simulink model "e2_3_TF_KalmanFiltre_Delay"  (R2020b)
settings: Solver=ode4  StartTime=0.0  StopTime=100  FixedStep=sampleTime  RelTol=1e-3  EnableMultiTasking=on
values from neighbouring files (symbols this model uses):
  k_d_x = 0.7    [startSimulation.m]
  k_d_y = 0.7    [startSimulation.m]
  k_d_yaw = 0.05    [startSimulation.m]
  k_d_z = 0.05    [startSimulation.m]
  k_i_x = 0.01    [startSimulation.m]
  k_i_y = 0.01    [startSimulation.m]
  k_i_yaw = 0.01    [startSimulation.m]
  k_i_z = 0.01    [startSimulation.m]
  k_p_x = 1    [startSimulation.m]
  k_p_y = 1    [startSimulation.m]
  k_p_yaw = 2    [startSimulation.m]
  k_p_z = 3    [startSimulation.m]
  saturation_psi = 2    [startSimulation.m]
  saturation_x = 2    [startSimulation.m]
  saturation_y = 2    [startSimulation.m]
  saturation_z = 2    [startSimulation.m]
undefined symbols (not defined in the file or in its folder): DiscIntNeverNeededParam, KiRollAttitude, sigbuilder_block
libraries: simulink x7, pid_lib x2, aerolibanimutils x1

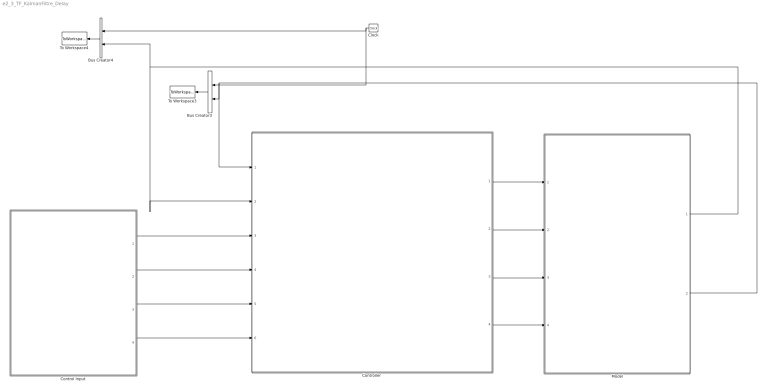
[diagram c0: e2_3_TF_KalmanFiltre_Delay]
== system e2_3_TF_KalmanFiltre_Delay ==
  Bus Creator3 : BusCreator  Inputs=2
  Bus Creator4 : BusCreator  Inputs=2
  Clock : Clock
  Control Input : Subsystem
  "Controller " : Subsystem
  Model : Subsystem
  To Workspace3 : ToWorkspace  VariableName=r1_pos_array  SampleTime=-1
  To Workspace4 : ToWorkspace  VariableName=r1_vel_array  SampleTime=-1
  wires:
  Clock/1 -> Bus Creator4/1, Bus Creator3/1
  Bus Creator3/1 -> To Workspace3/1
  Bus Creator4/1 -> To Workspace4/1
  "Controller "/1(Controller Output X) -> Model/1(Commande Input X)
  "Controller "/2(Controller Output Y) -> Model/2(Commande Input Y)
  "Controller "/3(Controller Output H) -> Model/3(Commande Input H)
  "Controller "/4(Controller Output Psi) -> Model/4(Commande Input Psi)
  Control Input/1(ux) -> "Controller "/3(Control input X)
  Control Input/2(uy) -> "Controller "/4(Control input Y)
  Control Input/3(uz) -> "Controller "/5(Control input H)
  Control Input/4(upsi) -> "Controller "/6(Control input Psi)
  Model/2(Output Position) -> "Controller "/1(Feedback Position), Bus Creator3/2
  Model/1(Output Velocity) -> "Controller "/2(Feedback Velocity), Bus Creator4/2

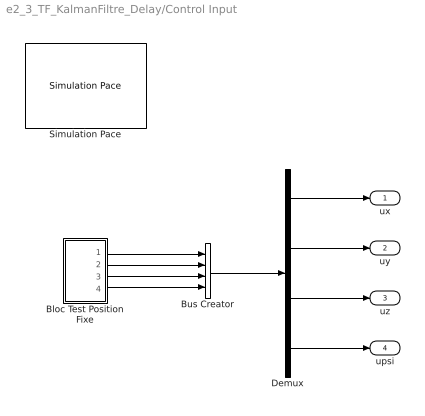
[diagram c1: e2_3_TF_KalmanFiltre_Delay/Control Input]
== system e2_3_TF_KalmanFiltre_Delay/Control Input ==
  Bloc Test Position Fixe : Subsystem
  Bus Creator : BusCreator  Inputs=4
  Demux : Demux
  Simulation Pace : aerolibanimutils/Simulation Pace  SimulationPace=100  SleepMode=MATLAB Thread  OutputPaceError=off  SampleTime=-1
  ux : Outport  VectorParamsAs1DForOutWhenUnconnected=off
  uy : Outport  Port=2  VectorParamsAs1DForOutWhenUnconnected=off
  uz : Outport  Port=3  VectorParamsAs1DForOutWhenUnconnected=off
  upsi : Outport  Port=4  VectorParamsAs1DForOutWhenUnconnected=off
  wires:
  Demux/2 -> uy/1
  Demux/1 -> ux/1
  Bloc Test Position Fixe/2(uy) -> Bus Creator/2
  Demux/3 -> uz/1
  Demux/4 -> upsi/1
  Bloc Test Position Fixe/4(upsi) -> Bus Creator/4
  Bloc Test Position Fixe/3(uz) -> Bus Creator/3
  Bloc Test Position Fixe/1(ux) -> Bus Creator/1
  Bus Creator/1 -> Demux/1

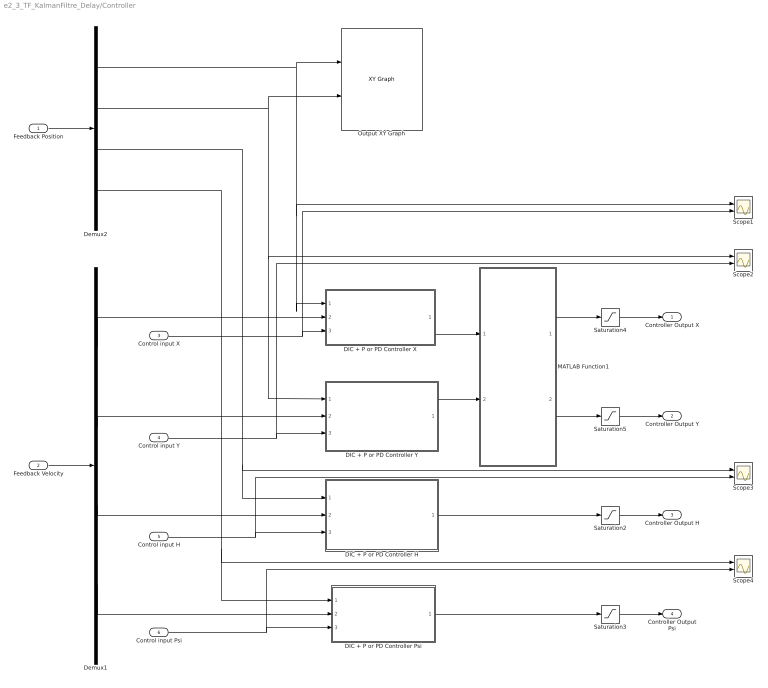
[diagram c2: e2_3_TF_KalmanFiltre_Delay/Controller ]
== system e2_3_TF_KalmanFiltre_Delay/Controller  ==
  Feedback Position : Inport
  Feedback Velocity : Inport  Port=2
  Control input X : Inport  Port=3
  Control input Y : Inport  Port=4
  Control input H : Inport  Port=5
  Control input Psi : Inport  Port=6
  DIC + P or PD Controller H : Subsystem
  DIC + P or PD Controller Psi : Subsystem
  DIC + P or PD Controller X : Subsystem
  DIC + P or PD Controller Y : Subsystem
  Demux1 : Demux
  Demux2 : Demux
  MATLAB Function1 : MATLAB Function  TreatAsAtomicUnit=on
  Output XY Graph : simulink/Sinks/XY Graph  Commented=on  xmin=-5  xmax=5  ymin=-5  ymax=5  st=-1
  Saturation2 : Saturate  UpperLimit=saturation_z  LowerLimit=-saturation_z
  Saturation3 : Saturate  UpperLimit=saturation_psi  LowerLimit=-saturation_psi
  Saturation4 : Saturate  UpperLimit=saturation_x  LowerLimit=-saturation_x
  Saturation5 : Saturate  UpperLimit=saturation_y  LowerLimit=-saturation_y
  Scope{1..4} (4 alike) : Scope  NumInputPorts=2
  Controller Output X : Outport  VectorParamsAs1DForOutWhenUnconnected=off
  Controller Output Y : Outport  Port=2  VectorParamsAs1DForOutWhenUnconnected=off
  Controller Output H : Outport  Port=3  VectorParamsAs1DForOutWhenUnconnected=off
  Controller Output Psi : Outport  Port=4  VectorParamsAs1DForOutWhenUnconnected=off
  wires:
  Feedback Position/1 -> Demux2/1
  Feedback Velocity/1 -> Demux1/1
  Demux1/2 -> DIC + P or PD Controller Y/2(Feedback Velocity Y)
  Demux2/3 -> Scope3/1, DIC + P or PD Controller H/1(Feedback Position H)
  Demux1/1 -> DIC + P or PD Controller X/2(Feedback Velocity X)
  Demux1/3 -> DIC + P or PD Controller H/2(Feedback Velocity H)
  Control input X/1 -> Scope1/2, DIC + P or PD Controller X/3(Control Input X)
  Control input H/1 -> Scope3/2, DIC + P or PD Controller H/3(Control Input H)
  Saturation4/1 -> Controller Output X/1
  Saturation5/1 -> Controller Output Y/1
  Saturation2/1 -> Controller Output H/1
  Saturation3/1 -> Controller Output Psi/1
  Control input Y/1 -> Scope2/2, DIC + P or PD Controller Y/3(Control Input Y)
  DIC + P or PD Controller H/1(Controller Output H) -> Saturation2/1
  DIC + P or PD Controller Psi/1(Controller Output Psi) -> Saturation3/1
  Demux2/1 -> Scope1/1, DIC + P or PD Controller X/1(Feedback Position X), Output XY Graph/1
  Demux2/2 -> Scope2/1, DIC + P or PD Controller Y/1(Feedback Position Y), Output XY Graph/2
  Demux2/4 -> Scope4/1, DIC + P or PD Controller Psi/1(Feedback Position Psi)
  Demux1/4 -> DIC + P or PD Controller Psi/2(Feedback Velocity Psi)
  Control input Psi/1 -> Scope4/2, DIC + P or PD Controller Psi/3(Control input Psi)
  MATLAB Function1/2(phi) -> Saturation5/1
  MATLAB Function1/1(theta) -> Saturation4/1
  DIC + P or PD Controller X/1(Controller Output X) -> MATLAB Function1/1(eax)
  DIC + P or PD Controller Y/1(Controller Output Y) -> MATLAB Function1/2(eay)

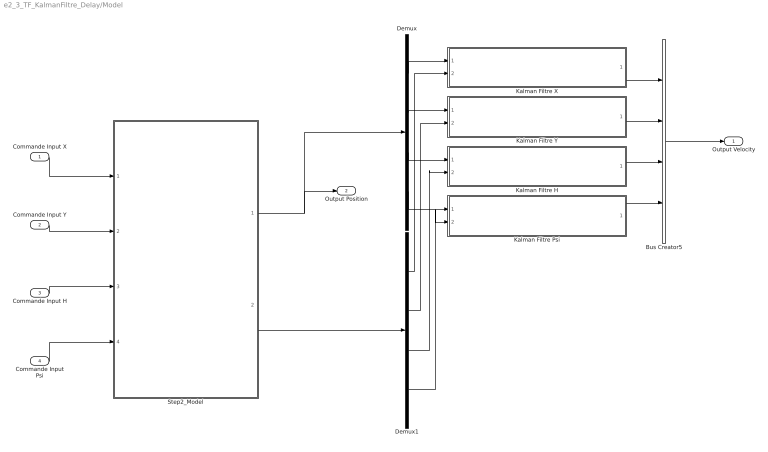
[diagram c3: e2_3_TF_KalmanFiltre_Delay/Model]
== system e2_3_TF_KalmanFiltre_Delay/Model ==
  Commande Input X : Inport
  Commande Input Y : Inport  Port=2
  Commande Input H : Inport  Port=3
  Commande Input Psi : Inport  Port=4
  Bus Creator5 : BusCreator  Inputs=4
  Demux : Demux
  Demux1 : Demux
  Kalman Filtre H : Subsystem
  Kalman Filtre Psi : Subsystem
  Kalman Filtre X : Subsystem
  Kalman Filtre Y : Subsystem
  Step2_Model : Subsystem
  Output Velocity : Outport  VectorParamsAs1DForOutWhenUnconnected=off
  Output Position : Outport  Port=2  VectorParamsAs1DForOutWhenUnconnected=off
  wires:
  Demux/4 -> Kalman Filtre Psi/1(The system output: Position)
  Bus Creator5/1 -> Output Velocity/1
  Demux/1 -> Kalman Filtre X/1(The system output: Position)
  Kalman Filtre X/1(Out velocity feedback) -> Bus Creator5/1
  Kalman Filtre Psi/1(Out velocity feedback) -> Bus Creator5/4
  Demux/2 -> Kalman Filtre Y/1(The system output: Position)
  Kalman Filtre Y/1(Out velocity feedback) -> Bus Creator5/2
  Kalman Filtre H/1(Out velocity feedback) -> Bus Creator5/3
  Demux/3 -> Kalman Filtre H/1(The system output: Position)
  Demux1/1 -> Kalman Filtre X/2(In2)
  Demux1/2 -> Kalman Filtre Y/2(In2)
  Demux1/3 -> Kalman Filtre H/2(In2)
  Demux1/4 -> Kalman Filtre Psi/2(In2)
  Commande Input H/1 -> Step2_Model/3(In3)
  Step2_Model/1(Position) -> Output Position/1, Demux/1
  Commande Input Psi/1 -> Step2_Model/4(In4)
  Commande Input X/1 -> Step2_Model/1(In1)
  Commande Input Y/1 -> Step2_Model/2(In2)
  Step2_Model/2(Velocity) -> Demux1/1

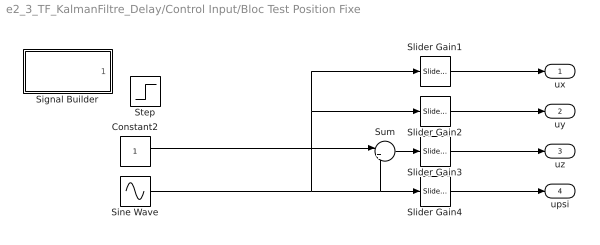
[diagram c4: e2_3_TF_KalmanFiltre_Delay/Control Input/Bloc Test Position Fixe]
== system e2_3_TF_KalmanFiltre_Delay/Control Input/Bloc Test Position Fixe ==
  Constant2 : Constant
  Signal Builder : Subsystem  Tag=STV Subsys  LoadFcn=sigbuilder_block('load');  StartFcn=sigbuilder_block('start');  StopFcn=sigbuilder_block('stop');  ClipboardFcn=sigbuilder_block('clipboard');  mask(Sigbuilder block){tuvar=[0:10]}
      mask help: Simulink:masks:SigbuilderBlock_MD
      mask init:
      | if ~strcmp(get_param(bdroot(gcbh),'SimulationStatus'),'stopped') tuvar = sigbuilder_block('maskInit'); end
  Sine Wave : Sin  Frequency=0.5  SampleTime=0
  Slider Gain1 : simulink/Math Operations/Slider Gain  gain=1  low=-10  high=10
  Slider Gain2 : simulink/Math Operations/Slider Gain  gain=0  low=-10  high=10
  Slider Gain3 : simulink/Math Operations/Slider Gain  gain=1  low=-2  high=2
  Slider Gain4 : simulink/Math Operations/Slider Gain  gain=0  low=-2  high=2
  Step : Step  Time=5  SampleTime=0
  Sum : Sum  Inputs=|++
  ux : Outport  VectorParamsAs1DForOutWhenUnconnected=off
  uy : Outport  Port=2  VectorParamsAs1DForOutWhenUnconnected=off
  uz : Outport  Port=3  VectorParamsAs1DForOutWhenUnconnected=off
  upsi : Outport  Port=4  VectorParamsAs1DForOutWhenUnconnected=off
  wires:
  Slider Gain1/1 -> ux/1
  Slider Gain2/1 -> uy/1
  Slider Gain3/1 -> uz/1
  Slider Gain4/1 -> upsi/1
  Sum/1 -> Slider Gain3/1
  Constant2/1 -> Sum/1
  Sine Wave/1 -> Slider Gain2/1, Slider Gain1/1, Sum/2, Slider Gain4/1

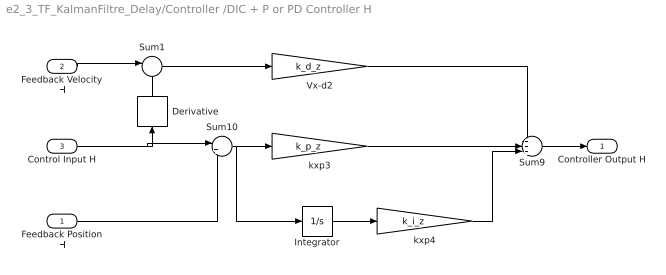
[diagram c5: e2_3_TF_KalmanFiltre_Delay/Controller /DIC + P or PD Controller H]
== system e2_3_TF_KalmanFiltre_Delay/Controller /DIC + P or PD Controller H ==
  Feedback Position H : Inport
  Feedback Velocity H : Inport  Port=2
  Control Input H : Inport  Port=3
  Derivative : Derivative
  Integrator : Integrator
  Sum1 : Sum  Inputs=|-+
  Sum10 : Sum  Inputs=|+-
  Sum9 : Sum  Inputs=+++|
  Vx-d2 : Gain  Gain=k_d_z
  kxp3 : Gain  Gain=k_p_z
  kxp4 : Gain  Gain=k_i_z
  Controller Output H : Outport  VectorParamsAs1DForOutWhenUnconnected=off
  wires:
  Sum9/1 -> Controller Output H/1
  Sum10/1 -> kxp3/1, Integrator/1
  kxp3/1 -> Sum9/2
  Vx-d2/1 -> Sum9/1
  Feedback Velocity H/1 -> Sum1/1
  Sum1/1 -> Vx-d2/1
  Integrator/1 -> kxp4/1
  kxp4/1 -> Sum9/3
  Control Input H/1 -> Sum10/1, Derivative/1
  Feedback Position H/1 -> Sum10/2
  Derivative/1 -> Sum1/2

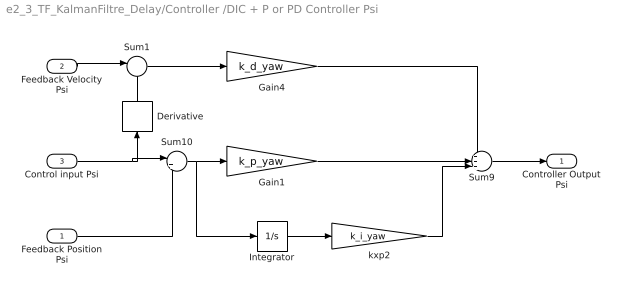
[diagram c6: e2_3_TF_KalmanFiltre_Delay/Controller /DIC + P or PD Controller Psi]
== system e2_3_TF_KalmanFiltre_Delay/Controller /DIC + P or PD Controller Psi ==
  Feedback Position Psi : Inport
  Feedback Velocity Psi : Inport  Port=2
  Control input Psi : Inport  Port=3
  Derivative : Derivative
  Gain1 : Gain  Gain=k_p_yaw
  Gain4 : Gain  Gain=k_d_yaw
  Integrator : Integrator
  Sum1 : Sum  Inputs=|-+
  Sum10 : Sum  Inputs=|+-
  Sum9 : Sum  Inputs=+++|
  kxp2 : Gain  Gain=k_i_yaw
  Controller Output Psi : Outport  VectorParamsAs1DForOutWhenUnconnected=off
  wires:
  Sum9/1 -> Controller Output Psi/1
  kxp2/1 -> Sum9/3
  Control input Psi/1 -> Sum10/1, Derivative/1
  Gain4/1 -> Sum9/1
  Sum10/1 -> Gain1/1, Integrator/1
  Integrator/1 -> kxp2/1
  Feedback Velocity Psi/1 -> Sum1/1
  Sum1/1 -> Gain4/1
  Gain1/1 -> Sum9/2
  Derivative/1 -> Sum1/2
  Feedback Position Psi/1 -> Sum10/2

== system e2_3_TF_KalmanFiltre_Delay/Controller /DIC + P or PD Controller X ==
  Feedback Position X : Inport
  Feedback Velocity X : Inport  Port=2
  Control Input X : Inport  Port=3
  PID1 : Subsystem
  Sum3 : Sum  Inputs=|+-
  Sum4 : Sum  Inputs=|+-
  roll_attitude2 : pid_lib/PID Controller  Controller=P  Form=Parallel  TimeDomain=Discrete-time  UseExternalTs=off  SampleTime=-1  IntegratorMethod=Forward Euler  FilterMethod=Forward Euler  ControllerParametersSource=internal  P=1  I=KiRollAttitude  D=0.01  UseFilter=on  N=100  TunerSelectOption=Transfer Function Based (PID Tuner App)  InitialConditionSource=internal  InitialConditionForIntegrator=0  InitialConditionForFilter=0  DifferentiatorICPrevScaledInput=0  ExternalReset=none  TrackingMode=off  Kt=1  LimitOutput=on  SatLimitsSource=internal  UpperSaturationLimit=100  LowerSaturationLimit=-100  LinearizeAsGain=on  AntiWindupMode=back-calculation  Kb=1  POutMin=[]  POutMax=[]  IOutMin=[]  IOutMax=[]  DOutMin=[]  DOutMax=[]  NOutMin=[]  NOutMax=[]  SumOutMin=[]  SumOutMax=[]  SaturationOutMin=[]  SaturationOutMax=[]  PParamMin=[]  PParamMax=[]  IParamMin=[]  IParamMax=[]  DParamMin=[]  DParamMax=[]  NParamMin=[]  NParamMax=[]  KbParamMin=[]  KbParamMax=[]  KtParamMin=[]  KtParamMax=[]  KbOutMin=[]  KbOutMax=[]  KtOutMin=[]  KtOutMax=[]  IntegratorOutMin=[]  IntegratorOutMax=[]  FilterOutMin=[]  FilterOutMax=[]  SumI1OutMin=[]  SumI1OutMax=[]  SumI2OutMin=[]  SumI2OutMax=[]  SumI3OutMin=[]  SumI3OutMax=[]  SumI4OutMin=[]  SumI4OutMax=[]  SumDOutMin=[]  SumDOutMax=[]  DifferentiatorOutMin=[]  DifferentiatorOutMax=[]  FilterDiffOutCoefMin=[]  FilterDiffOutCoefMax=[]  ReciprocalOutMin=[]  ReciprocalOutMax=[]  SumDenOutMin=[]  SumDenOutMax=[]  SumNumOutMin=[]  SumNumOutMax=[]  DivideOutMin=[]  DivideOutMax=[]  UdiffTsProdOutMin=[]  UdiffTsProdOutMax=[]  NTsProdOutMin=[]  NTsProdOutMax=[]  UintegralTsProdOutMin=[]  UintegralTsProdOutMax=[]  UngainTsProdOutMin=[]  UngainTsProdOutMax=[]  IntegratorContinuousStateAttributes=''  IntegratorStateMustResolveToSignalObject=off  IntegratorRTWStateStorageClass=Auto  FilterContinuousStateAttributes=''  FilterStateMustResolveToSignalObject=off  FilterRTWStateStorageClass=Auto  ParallelPVariant=InternalParameters  IdealPVariant=Disabled  IVariant=Disabled  DVariant=Disabled  IntegratorVariant=Disabled  SatVariant=Enabled  AWVariant=Disabled  PCopyVariant=Disabled  TRVariant=Disabled  FdbkBlocksVariant=Forward  IdealPFdbkVariant=Disabled  SatFdbkVariant=Disabled  DerivativeFilterVariant=Disabled  NVariant=Disabled  NCopyVariant=Disabled_SignalSpec  FilterICVariant=Disabled  IntegratorICVariant=Disabled  ExternalResetVariant=Disabled  TRSumVariant=Passthrough  SumFdbkVariant=Disabled  SumVariant=Passthrough_P  TsampFilterVariant=InternalTs  TsampNgainVariant=Passthrough  TsampIntegralVariant=Disabled_SignalSpec  ExternalSaturationOutDataTypeStr=Inherit: Same as second input
  Controller Output X : Outport  VectorParamsAs1DForOutWhenUnconnected=off
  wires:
  roll_attitude2/1 -> Sum4/1
  Sum3/1 -> roll_attitude2/1
  Sum4/1 -> PID1/1(x)
  PID1/1(y) -> Controller Output X/1
  Feedback Velocity X/1 -> Sum4/2
  Control Input X/1 -> Sum3/1
  Feedback Position X/1 -> Sum3/2

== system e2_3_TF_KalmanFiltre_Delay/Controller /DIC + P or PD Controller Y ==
  Feedback Position Y : Inport
  Feedback Velocity Y : Inport  Port=2
  Control Input Y : Inport  Port=3
  PID2 : Subsystem
  Sum : Sum  Inputs=|+-
  Sum2 : Sum  Inputs=|+-
  roll_attitude : pid_lib/PID Controller  Controller=P  Form=Parallel  TimeDomain=Discrete-time  UseExternalTs=off  SampleTime=-1  IntegratorMethod=Forward Euler  FilterMethod=Forward Euler  ControllerParametersSource=internal  P=1  I=KiRollAttitude  D=0.01  UseFilter=on  N=100  TunerSelectOption=Transfer Function Based (PID Tuner App)  InitialConditionSource=internal  InitialConditionForIntegrator=0  InitialConditionForFilter=0  DifferentiatorICPrevScaledInput=0  ExternalReset=none  TrackingMode=off  Kt=1  LimitOutput=on  SatLimitsSource=internal  UpperSaturationLimit=1  LowerSaturationLimit=-1  LinearizeAsGain=on  AntiWindupMode=back-calculation  Kb=1  POutMin=[]  POutMax=[]  IOutMin=[]  IOutMax=[]  DOutMin=[]  DOutMax=[]  NOutMin=[]  NOutMax=[]  SumOutMin=[]  SumOutMax=[]  SaturationOutMin=[]  SaturationOutMax=[]  PParamMin=[]  PParamMax=[]  IParamMin=[]  IParamMax=[]  DParamMin=[]  DParamMax=[]  NParamMin=[]  NParamMax=[]  KbParamMin=[]  KbParamMax=[]  KtParamMin=[]  KtParamMax=[]  KbOutMin=[]  KbOutMax=[]  KtOutMin=[]  KtOutMax=[]  IntegratorOutMin=[]  IntegratorOutMax=[]  FilterOutMin=[]  FilterOutMax=[]  SumI1OutMin=[]  SumI1OutMax=[]  SumI2OutMin=[]  SumI2OutMax=[]  SumI3OutMin=[]  SumI3OutMax=[]  SumI4OutMin=[]  SumI4OutMax=[]  SumDOutMin=[]  SumDOutMax=[]  DifferentiatorOutMin=[]  DifferentiatorOutMax=[]  FilterDiffOutCoefMin=[]  FilterDiffOutCoefMax=[]  ReciprocalOutMin=[]  ReciprocalOutMax=[]  SumDenOutMin=[]  SumDenOutMax=[]  SumNumOutMin=[]  SumNumOutMax=[]  DivideOutMin=[]  DivideOutMax=[]  UdiffTsProdOutMin=[]  UdiffTsProdOutMax=[]  NTsProdOutMin=[]  NTsProdOutMax=[]  UintegralTsProdOutMin=[]  UintegralTsProdOutMax=[]  UngainTsProdOutMin=[]  UngainTsProdOutMax=[]  IntegratorContinuousStateAttributes=''  IntegratorStateMustResolveToSignalObject=off  IntegratorRTWStateStorageClass=Auto  FilterContinuousStateAttributes=''  FilterStateMustResolveToSignalObject=off  FilterRTWStateStorageClass=Auto  ParallelPVariant=InternalParameters  IdealPVariant=Disabled  IVariant=Disabled  DVariant=Disabled  IntegratorVariant=Disabled  SatVariant=Enabled  AWVariant=Disabled  PCopyVariant=Disabled  TRVariant=Disabled  FdbkBlocksVariant=Forward  IdealPFdbkVariant=Disabled  SatFdbkVariant=Disabled  DerivativeFilterVariant=Disabled  NVariant=Disabled  NCopyVariant=Disabled_SignalSpec  FilterICVariant=Disabled  IntegratorICVariant=Disabled  ExternalResetVariant=Disabled  TRSumVariant=Passthrough  SumFdbkVariant=Disabled  SumVariant=Passthrough_P  TsampFilterVariant=InternalTs  TsampNgainVariant=Passthrough  TsampIntegralVariant=Disabled_SignalSpec  ExternalSaturationOutDataTypeStr=Inherit: Same as second input
  Controller Output Y : Outport  VectorParamsAs1DForOutWhenUnconnected=off
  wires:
  Sum/1 -> roll_attitude/1
  roll_attitude/1 -> Sum2/1
  Sum2/1 -> PID2/1(x)
  Feedback Position Y/1 -> Sum/2
  Feedback Velocity Y/1 -> Sum2/2
  Control Input Y/1 -> Sum/1
  PID2/1(y) -> Controller Output Y/1

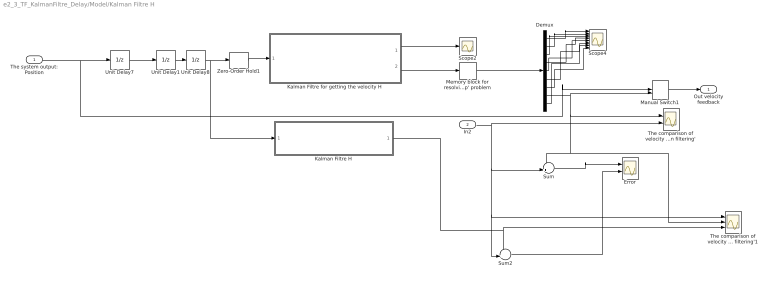
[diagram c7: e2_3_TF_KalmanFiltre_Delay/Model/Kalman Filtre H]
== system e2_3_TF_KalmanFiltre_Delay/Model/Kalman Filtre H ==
  The system output: Position : Inport
  In2 : Inport  Port=2
  Demux : Demux  Outputs=9
  Error : Scope  NumInputPorts=2
  Kalman Filtre H : Subsystem
  Kalman Filtre for getting the velocity H : MATLAB Function  TreatAsAtomicUnit=on  SystemSampleTime=0.01
  Manual Switch1 : ManualSwitch  CurrentSetting=0
  Memory block for resolving the 'algebraic loop' problem : Memory
  Scope2 : Scope
  Scope4 : Scope  NumInputPorts=8
  Sum : Sum  Inputs=-+|
  Sum2 : Sum  Inputs=-+|
  The comparison of velocity signal between 'Derivative' and 'Kalman filtering' : Scope  NumInputPorts=2
  The comparison of velocity signal between 'Derivative' and 'Kalman filtering'1 : Scope  NumInputPorts=3
  Unit Delay1 : UnitDelay  SampleTime=-1  HasFrameUpgradeWarning=on
  Unit Delay7 : UnitDelay  SampleTime=-1  HasFrameUpgradeWarning=on
  Unit Delay8 : UnitDelay  SampleTime=-1  HasFrameUpgradeWarning=on
  Zero-Order Hold1 : ZeroOrderHold  SampleTime=-1
  Out velocity feedback : Outport  VectorParamsAs1DForOutWhenUnconnected=off
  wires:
  Kalman Filtre for getting the velocity H/1(Covariance_matrice) -> Scope2/1
  Kalman Filtre for getting the velocity H/2(X_Kalmanfiltred) -> Memory block for resolving the 'algebraic loop' problem/1
  Memory block for resolving the 'algebraic loop' problem/1 -> Demux/1
  Zero-Order Hold1/1 -> Kalman Filtre for getting the velocity H/1(Mesurement_Velocity)
  Manual Switch1/1 -> Out velocity feedback/1
  Demux/1 -> Scope4/1
  The system output: Position/1 -> Unit Delay7/1, Manual Switch1/1
  Demux/2 -> Scope4/2
  Demux/3 -> Scope4/3
  Demux/4 -> Scope4/4
  Demux/5 -> Scope4/5
  Unit Delay8/1 -> Kalman Filtre H/1(The system output: Position), Zero-Order Hold1/1
  Demux/6 -> Scope4/6
  Demux/7 -> Scope4/8
  Demux/8 -> The comparison of velocity signal between 'Derivative' and 'Kalman filtering'1/2, Sum/1, The comparison of velocity signal between 'Derivative' and 'Kalman filtering'/1, Manual Switch1/2
  Demux/9 -> Scope4/7
  In2/1 -> The comparison of velocity signal between 'Derivative' and 'Kalman filtering'/2, Sum2/2, The comparison of velocity signal between 'Derivative' and 'Kalman filtering'1/1, Sum/2
  Unit Delay7/1 -> Unit Delay1/1
  Unit Delay1/1 -> Unit Delay8/1
  Sum/1 -> Error/1
  Kalman Filtre H/1(Out velocity feedback) -> Sum2/1, The comparison of velocity signal between 'Derivative' and 'Kalman filtering'1/3
  Sum2/1 -> Error/2

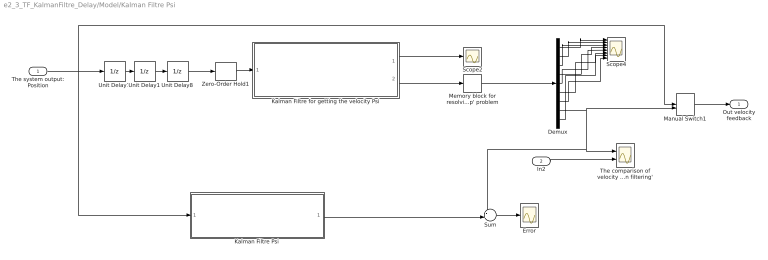
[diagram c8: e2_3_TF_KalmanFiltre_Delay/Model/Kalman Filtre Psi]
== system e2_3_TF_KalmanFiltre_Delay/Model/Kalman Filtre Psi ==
  The system output: Position : Inport
  In2 : Inport  Port=2
  Demux : Demux  Outputs=9
  Error : Scope
  Kalman Filtre Psi : Subsystem
  Kalman Filtre for getting the velocity Psi : MATLAB Function  TreatAsAtomicUnit=on  SystemSampleTime=0.01
  Manual Switch1 : ManualSwitch  CurrentSetting=0
  Memory block for resolving the 'algebraic loop' problem : Memory
  Scope2 : Scope
  Scope4 : Scope  NumInputPorts=8
  Sum : Sum  Inputs=-+|
  The comparison of velocity signal between 'Derivative' and 'Kalman filtering' : Scope  NumInputPorts=2
  Unit Delay1 : UnitDelay  SampleTime=-1  HasFrameUpgradeWarning=on
  Unit Delay7 : UnitDelay  SampleTime=-1  HasFrameUpgradeWarning=on
  Unit Delay8 : UnitDelay  SampleTime=-1  HasFrameUpgradeWarning=on
  Zero-Order Hold1 : ZeroOrderHold  SampleTime=-1
  Out velocity feedback : Outport  VectorParamsAs1DForOutWhenUnconnected=off
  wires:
  Kalman Filtre for getting the velocity Psi/1(Covariance_matrice) -> Scope2/1
  Kalman Filtre for getting the velocity Psi/2(X_Kalmanfiltred) -> Memory block for resolving the 'algebraic loop' problem/1
  Memory block for resolving the 'algebraic loop' problem/1 -> Demux/1
  Zero-Order Hold1/1 -> Kalman Filtre for getting the velocity Psi/1(Mesurement_Velocity)
  Manual Switch1/1 -> Out velocity feedback/1
  Demux/1 -> Scope4/1
  The system output: Position/1 -> Kalman Filtre Psi/1(The system output: Position), Manual Switch1/1, Unit Delay7/1
  Demux/2 -> Scope4/2
  Demux/3 -> Scope4/3
  Demux/4 -> Scope4/4
  Demux/5 -> Scope4/5
  Unit Delay8/1 -> Zero-Order Hold1/1
  Demux/6 -> Scope4/6
  Demux/7 -> Scope4/8
  Demux/8 -> Sum/1, The comparison of velocity signal between 'Derivative' and 'Kalman filtering'/1, Manual Switch1/2
  Demux/9 -> Scope4/7
  In2/1 -> The comparison of velocity signal between 'Derivative' and 'Kalman filtering'/2
  Unit Delay7/1 -> Unit Delay1/1
  Unit Delay1/1 -> Unit Delay8/1
  Sum/1 -> Error/1
  Kalman Filtre Psi/1(Out velocity feedback) -> Sum/2

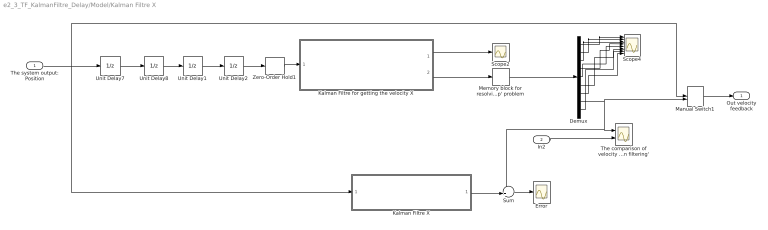
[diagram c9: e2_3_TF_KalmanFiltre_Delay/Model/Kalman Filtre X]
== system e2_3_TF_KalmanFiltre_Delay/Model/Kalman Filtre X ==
  The system output: Position : Inport
  In2 : Inport  Port=2
  Demux : Demux  Outputs=9
  Error : Scope
  Kalman Filtre X : Subsystem
  Kalman Filtre for getting the velocity X : MATLAB Function  TreatAsAtomicUnit=on  SystemSampleTime=0.01
  Manual Switch1 : ManualSwitch  CurrentSetting=0
  Memory block for resolving the 'algebraic loop' problem : Memory
  Scope2 : Scope
  Scope4 : Scope  NumInputPorts=8
  Sum : Sum  Inputs=-+|
  The comparison of velocity signal between 'Derivative' and 'Kalman filtering' : Scope  NumInputPorts=2
  Unit Delay{1..2,7..8} (4 alike) : UnitDelay  SampleTime=-1  HasFrameUpgradeWarning=on
  Zero-Order Hold1 : ZeroOrderHold  SampleTime=-1
  Out velocity feedback : Outport  VectorParamsAs1DForOutWhenUnconnected=off
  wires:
  Kalman Filtre for getting the velocity X/1(Covariance_matrice) -> Scope2/1
  Kalman Filtre for getting the velocity X/2(X_Kalmanfiltred) -> Memory block for resolving the 'algebraic loop' problem/1
  Memory block for resolving the 'algebraic loop' problem/1 -> Demux/1
  Zero-Order Hold1/1 -> Kalman Filtre for getting the velocity X/1(Mesurement_Velocity)
  Manual Switch1/1 -> Out velocity feedback/1
  Demux/1 -> Scope4/1
  The system output: Position/1 -> Kalman Filtre X/1(The system output: Position), Manual Switch1/1, Unit Delay7/1
  Demux/2 -> Scope4/2
  Demux/3 -> Scope4/3
  Demux/4 -> Scope4/4
  Demux/5 -> Scope4/5
  Unit Delay7/1 -> Unit Delay8/1
  Unit Delay8/1 -> Unit Delay1/1
  Demux/6 -> Scope4/6
  Demux/7 -> Scope4/8
  Demux/8 -> Sum/1, The comparison of velocity signal between 'Derivative' and 'Kalman filtering'/1, Manual Switch1/2
  Demux/9 -> Scope4/7
  In2/1 -> The comparison of velocity signal between 'Derivative' and 'Kalman filtering'/2
  Unit Delay1/1 -> Unit Delay2/1
  Unit Delay2/1 -> Zero-Order Hold1/1
  Kalman Filtre X/1(Out velocity feedback) -> Sum/2
  Sum/1 -> Error/1

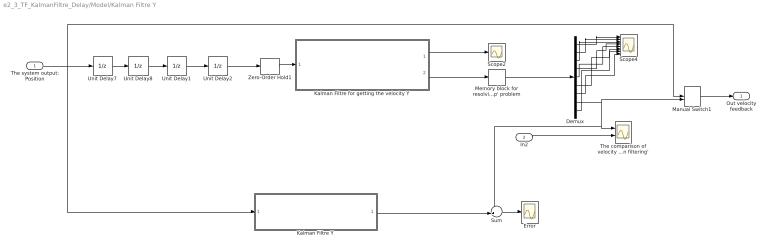
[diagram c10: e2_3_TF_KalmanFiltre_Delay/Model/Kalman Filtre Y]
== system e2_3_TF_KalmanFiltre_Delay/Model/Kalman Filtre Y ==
  The system output: Position : Inport
  In2 : Inport  Port=2
  Demux : Demux  Outputs=9
  Error : Scope
  Kalman Filtre Y : Subsystem
  Kalman Filtre for getting the velocity Y : MATLAB Function  TreatAsAtomicUnit=on  SystemSampleTime=0.01
  Manual Switch1 : ManualSwitch  CurrentSetting=0
  Memory block for resolving the 'algebraic loop' problem : Memory
  Scope2 : Scope
  Scope4 : Scope  NumInputPorts=8
  Sum : Sum  Inputs=-+|
  The comparison of velocity signal between 'Derivative' and 'Kalman filtering' : Scope  NumInputPorts=2
  Unit Delay{1..2,7..8} (4 alike) : UnitDelay  SampleTime=-1  HasFrameUpgradeWarning=on
  Zero-Order Hold1 : ZeroOrderHold  SampleTime=-1
  Out velocity feedback : Outport  VectorParamsAs1DForOutWhenUnconnected=off
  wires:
  Kalman Filtre for getting the velocity Y/1(Covariance_matrice) -> Scope2/1
  Kalman Filtre for getting the velocity Y/2(X_Kalmanfiltred) -> Memory block for resolving the 'algebraic loop' problem/1
  Memory block for resolving the 'algebraic loop' problem/1 -> Demux/1
  Zero-Order Hold1/1 -> Kalman Filtre for getting the velocity Y/1(Mesurement_Velocity)
  Manual Switch1/1 -> Out velocity feedback/1
  Demux/1 -> Scope4/1
  The system output: Position/1 -> Kalman Filtre Y/1(The system output: Position), Unit Delay7/1, Manual Switch1/1
  Demux/2 -> Scope4/2
  Demux/3 -> Scope4/3
  Demux/4 -> Scope4/4
  Demux/5 -> Scope4/5
  Unit Delay2/1 -> Zero-Order Hold1/1
  Demux/6 -> Scope4/6
  Demux/7 -> Scope4/8
  Demux/8 -> Sum/1, The comparison of velocity signal between 'Derivative' and 'Kalman filtering'/1, Manual Switch1/2
  Demux/9 -> Scope4/7
  In2/1 -> The comparison of velocity signal between 'Derivative' and 'Kalman filtering'/2
  Unit Delay1/1 -> Unit Delay2/1
  Unit Delay8/1 -> Unit Delay1/1
  Unit Delay7/1 -> Unit Delay8/1
  Sum/1 -> Error/1
  Kalman Filtre Y/1(Out velocity feedback) -> Sum/2

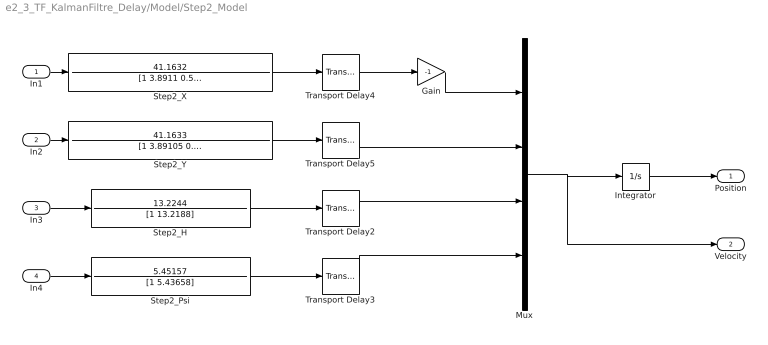
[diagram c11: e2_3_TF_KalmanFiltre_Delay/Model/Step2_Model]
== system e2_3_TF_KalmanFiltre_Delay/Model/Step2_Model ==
  In1 : Inport
  In2 : Inport  Port=2
  In3 : Inport  Port=3
  In4 : Inport  Port=4
  Gain : Gain  Gain=-1
  Integrator : Integrator
  Mux : Mux
  Step2_H : TransferFcn  Numerator=13.2244  Denominator=[1 13.2188]
  Step2_Psi : TransferFcn  Numerator=5.45157  Denominator=[1 5.43658]
  Step2_X : TransferFcn  Numerator=41.1632  Denominator=[1 3.8911 0.529635]
  Step2_Y : TransferFcn  Numerator=41.1633  Denominator=[1 3.89105 0.529839]
  Transport Delay2 : TransportDelay  DelayTime=0.0344
  Transport Delay3 : TransportDelay  DelayTime=0.0313
  Transport Delay4 : TransportDelay  DelayTime=0.0289
  Transport Delay5 : TransportDelay  DelayTime=0.0289
  Position : Outport  VectorParamsAs1DForOutWhenUnconnected=off
  Velocity : Outport  Port=2  VectorParamsAs1DForOutWhenUnconnected=off
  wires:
  Transport Delay2/1 -> Mux/3
  In2/1 -> Step2_Y/1
  In4/1 -> Step2_Psi/1
  Transport Delay3/1 -> Mux/4
  In1/1 -> Step2_X/1
  In3/1 -> Step2_H/1
  Step2_H/1 -> Transport Delay2/1
  Step2_Y/1 -> Transport Delay5/1
  Step2_X/1 -> Transport Delay4/1
  Step2_Psi/1 -> Transport Delay3/1
  Transport Delay4/1 -> Gain/1
  Transport Delay5/1 -> Mux/2
  Integrator/1 -> Position/1
  Mux/1 -> Velocity/1, Integrator/1
  Gain/1 -> Mux/1

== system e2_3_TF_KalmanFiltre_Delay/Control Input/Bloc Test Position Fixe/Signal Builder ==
  Demux : Demux  Tag=STV Demux  Outputs=1
  FromWs : FromWorkspace  Tag=STV FromWs  VariableName=tuvar
  Signal 2 : Outport  Tag=STV Outport  VectorParamsAs1DForOutWhenUnconnected=off
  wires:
  FromWs/1 -> Demux/1
  Demux/1 -> Signal 2/1

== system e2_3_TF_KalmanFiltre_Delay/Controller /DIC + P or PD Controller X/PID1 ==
  x : Inport
  Discrete Derivative : simulink/Discrete/Discrete Derivative  gainval=1.0  ICPrevScaledInput=0.0  OutMin=-5  OutMax=5  OutDataType=fixdt(1, 16)  OutScaling=2^-10  DoSatur=off
  Discrete-Time Integrator : DiscreteIntegrator  SampleTime=-1  LimitOutput=on  UpperSaturationLimit=5  LowerSaturationLimit=-5  ICPrevOutput=DiscIntNeverNeededParam  ICPrevScaledInput=DiscIntNeverNeededParam
  Sum : Sum  Inputs=+++  OutMin=-10  OutMax=10
  Vx-d3 : Gain  Gain=k_d_x
  kxp2 : Gain  Gain=k_i_x
  kxp3 : Gain  Gain=k_p_x
  y : Outport  InitialOutput=0  VectorParamsAs1DForOutWhenUnconnected=off
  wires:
  x/1 -> Vx-d3/1, kxp2/1, kxp3/1
  kxp2/1 -> Discrete-Time Integrator/1
  Vx-d3/1 -> Discrete Derivative/1
  kxp3/1 -> Sum/1
  Sum/1 -> y/1
  Discrete Derivative/1 -> Sum/3
  Discrete-Time Integrator/1 -> Sum/2

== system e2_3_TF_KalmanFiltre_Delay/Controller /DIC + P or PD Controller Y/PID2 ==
  x : Inport
  Discrete Derivative : simulink/Discrete/Discrete Derivative  gainval=1.0  ICPrevScaledInput=0.0  OutMin=[]  OutMax=[]  OutDataType=fixdt(1, 16)  OutScaling=2^-10  DoSatur=off
  Discrete-Time Integrator : DiscreteIntegrator  SampleTime=-1  LimitOutput=on  UpperSaturationLimit=10  LowerSaturationLimit=-10  ICPrevOutput=DiscIntNeverNeededParam  ICPrevScaledInput=DiscIntNeverNeededParam
  Sum : Sum  Inputs=+++  OutMin=-10  OutMax=10
  Vx-d2 : Gain  Gain=k_d_y
  kxp2 : Gain  Gain=k_p_y
  kxp3 : Gain  Gain=k_i_y
  y : Outport  InitialOutput=0  VectorParamsAs1DForOutWhenUnconnected=off
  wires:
  x/1 -> kxp2/1, kxp3/1, Vx-d2/1
  kxp3/1 -> Discrete-Time Integrator/1
  Vx-d2/1 -> Discrete Derivative/1
  kxp2/1 -> Sum/1
  Sum/1 -> y/1
  Discrete Derivative/1 -> Sum/3
  Discrete-Time Integrator/1 -> Sum/2

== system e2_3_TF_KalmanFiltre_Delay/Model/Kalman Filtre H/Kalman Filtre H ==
  The system output: Position : Inport
  Demux : Demux  Outputs=3
  Kalman Filtre for getting the velocity H : MATLAB Function  TreatAsAtomicUnit=on  SystemSampleTime=0.01
  Memory block for resolving the 'algebraic loop' problem : Memory
  Scope2 : Scope
  Scope4 : Scope  NumInputPorts=2
  Out velocity feedback : Outport  VectorParamsAs1DForOutWhenUnconnected=off
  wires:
  Demux/2 -> Out velocity feedback/1
  Memory block for resolving the 'algebraic loop' problem/1 -> Demux/1
  Kalman Filtre for getting the velocity H/1(Covariance_matrice) -> Scope2/1
  The system output: Position/1 -> Kalman Filtre for getting the velocity H/1(Mesurement_Velocity)
  Demux/1 -> Scope4/1
  Kalman Filtre for getting the velocity H/2(X_Kalmanfiltred) -> Memory block for resolving the 'algebraic loop' problem/1
  Demux/3 -> Scope4/2

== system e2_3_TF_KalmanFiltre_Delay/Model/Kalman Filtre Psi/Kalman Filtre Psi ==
  The system output: Position : Inport
  Demux : Demux  Outputs=3
  Kalman Filtre for getting the velocity Psi : MATLAB Function  TreatAsAtomicUnit=on  SystemSampleTime=0.01
  Memory block for resolving the 'algebraic loop' problem : Memory
  Scope1 : Scope  NumInputPorts=2
  Scope2 : Scope
  Out velocity feedback : Outport  VectorParamsAs1DForOutWhenUnconnected=off
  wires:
  Demux/2 -> Out velocity feedback/1
  Kalman Filtre for getting the velocity Psi/1(Covariance_matrice) -> Scope2/1
  The system output: Position/1 -> Kalman Filtre for getting the velocity Psi/1(Mesurement_Velocity)
  Demux/1 -> Scope1/1
  Demux/3 -> Scope1/2
  Kalman Filtre for getting the velocity Psi/2(X_Kalmanfiltred) -> Memory block for resolving the 'algebraic loop' problem/1
  Memory block for resolving the 'algebraic loop' problem/1 -> Demux/1

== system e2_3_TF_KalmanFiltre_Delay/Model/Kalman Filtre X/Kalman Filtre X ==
  The system output: Position : Inport
  Demux : Demux  Outputs=3
  Kalman Filtre for getting the velocity X : MATLAB Function  TreatAsAtomicUnit=on  SystemSampleTime=0.01
  Memory block for resolving the 'algebraic loop' problem : Memory
  Scope2 : Scope
  Scope4 : Scope  NumInputPorts=2
  Out velocity feedback : Outport  VectorParamsAs1DForOutWhenUnconnected=off
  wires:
  Kalman Filtre for getting the velocity X/1(Covariance_matrice) -> Scope2/1
  Kalman Filtre for getting the velocity X/2(X_Kalmanfiltred) -> Memory block for resolving the 'algebraic loop' problem/1
  Memory block for resolving the 'algebraic loop' problem/1 -> Demux/1
  The system output: Position/1 -> Kalman Filtre for getting the velocity X/1(Mesurement_Velocity)
  Demux/2 -> Out velocity feedback/1
  Demux/1 -> Scope4/2
  Demux/3 -> Scope4/1

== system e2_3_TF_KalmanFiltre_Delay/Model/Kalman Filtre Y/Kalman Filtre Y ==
  The system output: Position : Inport
  Demux : Demux  Outputs=3
  Kalman Filtre for getting the velocity Y : MATLAB Function  TreatAsAtomicUnit=on  SystemSampleTime=0.01
  Memory block for resolving the 'algebraic loop' problem : Memory
  Scope2 : Scope
  Scope4 : Scope  NumInputPorts=2
  Out velocity feedback : Outport  VectorParamsAs1DForOutWhenUnconnected=off
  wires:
  Kalman Filtre for getting the velocity Y/2(X_Kalmanfiltred) -> Memory block for resolving the 'algebraic loop' problem/1
  Demux/2 -> Out velocity feedback/1
  Kalman Filtre for getting the velocity Y/1(Covariance_matrice) -> Scope2/1
  Memory block for resolving the 'algebraic loop' problem/1 -> Demux/1
  The system output: Position/1 -> Kalman Filtre for getting the velocity Y/1(Mesurement_Velocity)
  Demux/1 -> Scope4/1
  Demux/3 -> Scope4/2

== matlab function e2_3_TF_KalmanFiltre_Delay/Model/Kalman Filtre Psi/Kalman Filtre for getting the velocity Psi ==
function [Covariance_matrice,X_Kalmanfiltred] = fcn(Mesurement_Velocity) % Mesurement_State

% Persistent process for saving the last state and initilizing the variable
persistent P0_static;
if isempty(P0_static)
    P0_static=[[0.1,0 0;0,0.1,0;0 0 0.1] zeros(3) zeros(3) ;zeros(3) [0.1,0 0;0,0.1,0;0 0 0.1] zeros(3);zeros(3) zeros(3) [0.1,0 0;0,0.1,0;0 0 0.1]]; % the initilized matrice of estimated error
end

persistent Xkf_static;
if isempty(Xkf_static)
    Xkf_static=[0;0;0;0;0;0;0;0;0]; % the initilized state from Kalman Estimaton
end

% Determine the constants

% Simple time
Ts =0.01;

% Process Noise
p_var =0.05; % sigma
Q = eye(3)*p_var^2; % the covariance matrice of process noise
W=Q*randn(3,1);  % process noise
Q_delay=[Q zeros(3) zeros(3);zeros(3) Q zeros(3);zeros(3) zeros(3) Q];
% Mesurement Noise
m_var = 0.01; % sigma
R = [m_var^2 ];  % the covariance matrice of mesurement noise
V=R*randn; % mesurement noise
R_delay=R;
V_delay=R_delay*randn;
% Observation matrice
H=[1 0 0];
H_delay=[0 0 0 0 0 0 H];
% The indentity matrice
I=eye(3); 
I_delay=eye(9);

A=[1 Ts 0.5*(Ts^2);0 1 Ts;0 0 1];
A_delay=[A zeros(3) zeros(3);zeros(3) A zeros(3); zeros(3) zeros(3) A];
% Steady-State equation

% persistent X_real_static;
% if isempty(X_real_static)
%     X_real_static=[0;0]; % the initilized state from Kalman Estimaton
% end
% X_real_forward=X_real_static;
% X_real=A*X_real_forward+W;
% X_real_static=X_real;    
% Mesurement_Velocity=H_delay*(Mesurement_State)+V_delay;

%   Kalman Update process
    X_pre=A_delay*Xkf_static; % State estimation
    P_pre=A_delay*P0_static*A_delay'+Q_delay; % Covariance matrice estimation

    Kg=P_pre*H_delay'*inv(H_delay*P_pre*H_delay'+R_delay); % Kalman Gain calculation

    X_Kalmanfiltred=X_pre+Kg*(Mesurement_Velocity-H_delay*X_pre); % State estimation update
    Covariance_matrice=(I_delay-Kg*H_delay)*P_pre; % Covariance matrice estimation update

% update the value of the persistent variable for iterating the Kalman process
P0_static=Covariance_matrice;
Xkf_static=X_Kalmanfiltred;

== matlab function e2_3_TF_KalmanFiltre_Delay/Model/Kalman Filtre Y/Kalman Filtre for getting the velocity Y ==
function [Covariance_matrice,X_Kalmanfiltred] = fcn(Mesurement_Velocity) % Mesurement_State

% Persistent process for saving the last state and initilizing the variable
persistent P0_static;
if isempty(P0_static)
       P0_static=[[0.1,0 0;0,0.1,0;0 0 0.1] zeros(3) zeros(3) ;zeros(3) [0.1,0 0;0,0.1,0;0 0 0.1] zeros(3);zeros(3) zeros(3) [0.1,0 0;0,0.1,0;0 0 0.1]]; % the initilized matrice of estimated error 
end

persistent Xkf_static;
if isempty(Xkf_static)
    Xkf_static=[0;0;0;0;0;0;0;0;0]; % the initilized state from Kalman Estimaton
end

% Determine the constants

% Simple time
Ts =0.01;

% Process Noise
p_var =0.05; % sigma
Q = eye(3)*p_var^2; % the covariance matrice of process noise
W=Q*randn(3,1);  % process noise
Q_delay=[Q zeros(3) zeros(3);zeros(3) Q zeros(3);zeros(3) zeros(3) Q];
% Mesurement Noise
m_var = 0.01; % sigma
R = [m_var^2 ];  % the covariance matrice of mesurement noise
V=R*randn; % mesurement noise
R_delay=R;
V_delay=R_delay*randn;
% Observation matrice
H=[1 0 0];
H_delay=[0 0 0 0 0 0 H];
% The indentity matrice
I=eye(3); 
I_delay=eye(9);

A=[1 Ts 0.5*(Ts^2);0 1 Ts;0 0 1];
A_delay=[A zeros(3) zeros(3);zeros(3) A zeros(3); zeros(3) zeros(3) A];
% Steady-State equation

% persistent X_real_static;
% if isempty(X_real_static)
%     X_real_static=[0;0]; % the initilized state from Kalman Estimaton
% end
% X_real_forward=X_real_static;
% X_real=A*X_real_forward+W;
% X_real_static=X_real;    
% Mesurement_Velocity=H_delay*(Mesurement_State)+V_delay;

%   Kalman Update process
    X_pre=A_delay*Xkf_static; % State estimation
    P_pre=A_delay*P0_static*A_delay'+Q_delay; % Covariance matrice estimation

    Kg=P_pre*H_delay'*inv(H_delay*P_pre*H_delay'+R_delay); % Kalman Gain calculation

    X_Kalmanfiltred=X_pre+Kg*(Mesurement_Velocity-H_delay*X_pre); % State estimation update
    Covariance_matrice=(I_delay-Kg*H_delay)*P_pre; % Covariance matrice estimation update

% update the value of the persistent variable for iterating the Kalman process
P0_static=Covariance_matrice;
Xkf_static=X_Kalmanfiltred;

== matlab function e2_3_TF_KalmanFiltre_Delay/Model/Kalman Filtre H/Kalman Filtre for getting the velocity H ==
function [Covariance_matrice,X_Kalmanfiltred] = fcn(Mesurement_Velocity) % Mesurement_State

% Persistent process for saving the last state and initilizing the variable
persistent P0_static;
if isempty(P0_static)
    P0_static=[[0.1,0 0;0,0.1,0;0 0 0.1] zeros(3) zeros(3) ;zeros(3) [0.1,0 0;0,0.1,0;0 0 0.1] zeros(3);zeros(3) zeros(3) [0.1,0 0;0,0.1,0;0 0 0.1]]; % the initilized matrice of estimated error
end

persistent Xkf_static;
if isempty(Xkf_static)
    Xkf_static=[0;0;0;0;0;0;0;0;0]; % the initilized state from Kalman Estimaton
end

% Determine the constants

% Simple time
Ts =0.01;

% Process Noise
p_var =0.1; % sigma
Q = eye(3)*p_var^2; % the covariance matrice of process noise
W=Q*randn(3,1);  % process noise
Q_delay=[Q zeros(3) zeros(3);zeros(3) Q zeros(3);zeros(3) zeros(3) Q];
% Mesurement Noise
m_var = 0.01; % sigma
R = [m_var^2 ];  % the covariance matrice of mesurement noise
V=R*randn; % mesurement noise
R_delay=R;
V_delay=R_delay*randn;
% Observation matrice
H=[1 0 0];
H_delay=[0 0 0 0 0 0 H];
% The indentity matrice
I=eye(3); 
I_delay=eye(9);

A=[1 Ts 0.5*(Ts^2);0 1 Ts;0 0 1];
A_delay=[A zeros(3) zeros(3);zeros(3) A zeros(3); zeros(3) zeros(3) A];
% Steady-State equation

% persistent X_real_static;
% if isempty(X_real_static)
%     X_real_static=[0;0]; % the initilized state from Kalman Estimaton
% end
% X_real_forward=X_real_static;
% X_real=A*X_real_forward+W;
% X_real_static=X_real;    
% Mesurement_Velocity=H_delay*(Mesurement_State)+V_delay;

%   Kalman Update process
    X_pre=A_delay*Xkf_static; % State estimation
    P_pre=A_delay*P0_static*A_delay'+Q_delay; % Covariance matrice estimation

    Kg=P_pre*H_delay'*inv(H_delay*P_pre*H_delay'+R_delay); % Kalman Gain calculation

    X_Kalmanfiltred=X_pre+Kg*(Mesurement_Velocity-H_delay*X_pre); % State estimation update
    Covariance_matrice=(I_delay-Kg*H_delay)*P_pre; % Covariance matrice estimation update

% update the value of the persistent variable for iterating the Kalman process
P0_static=Covariance_matrice;
Xkf_static=X_Kalmanfiltred;

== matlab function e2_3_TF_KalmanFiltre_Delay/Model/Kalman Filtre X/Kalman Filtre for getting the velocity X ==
function [Covariance_matrice,X_Kalmanfiltred] = fcn(Mesurement_Velocity) % Mesurement_State

% Persistent process for saving the last state and initilizing the variable
persistent P0_static;
if isempty(P0_static)
    P0_static=[[0.1,0 0;0,0.1,0;0 0 0.1] zeros(3) zeros(3) ;zeros(3) [0.1,0 0;0,0.1,0;0 0 0.1] zeros(3);zeros(3) zeros(3) [0.1,0 0;0,0.1,0;0 0 0.1]]; % the initilized matrice of estimated error
end

persistent Xkf_static;
if isempty(Xkf_static)
    Xkf_static=[0;0;0;0;0;0;0;0;0]; % the initilized state from Kalman Estimaton
end

% Determine the constants

% Simple time
Ts =0.01;

% Process Noise
p_var =0.05; % sigma
Q = eye(3)*p_var^2; % the covariance matrice of process noise
W=Q*randn(3,1);  % process noise
Q_delay=[Q zeros(3) zeros(3);zeros(3) Q zeros(3);zeros(3) zeros(3) Q];
% Mesurement Noise
m_var = 0.01; % sigma
R = [m_var^2 ];  % the covariance matrice of mesurement noise
V=R*randn; % mesurement noise
R_delay=R;
V_delay=R_delay*randn;
% Observation matrice
H=[1 0 0];
H_delay=[0 0 0 0 0 0 H];
% The indentity matrice
I=eye(3); 
I_delay=eye(9);

A=[1 Ts 0.5*(Ts^2);0 1 Ts;0 0 1];
A_delay=[A zeros(3) zeros(3);zeros(3) A zeros(3); zeros(3) zeros(3) A];
% Steady-State equation

% persistent X_real_static;
% if isempty(X_real_static)
%     X_real_static=[0;0]; % the initilized state from Kalman Estimaton
% end
% X_real_forward=X_real_static;
% X_real=A*X_real_forward+W;
% X_real_static=X_real;    
% Mesurement_Velocity=H_delay*(Mesurement_State)+V_delay;

%   Kalman Update process
    X_pre=A_delay*Xkf_static; % State estimation
    P_pre=A_delay*P0_static*A_delay'+Q_delay; % Covariance matrice estimation

    Kg=P_pre*H_delay'*inv(H_delay*P_pre*H_delay'+R_delay); % Kalman Gain calculation

    X_Kalmanfiltred=X_pre+Kg*(Mesurement_Velocity-H_delay*X_pre); % State estimation update
    Covariance_matrice=(I_delay-Kg*H_delay)*P_pre; % Covariance matrice estimation update

% update the value of the persistent variable for iterating the Kalman process
P0_static=Covariance_matrice;
Xkf_static=X_Kalmanfiltred;

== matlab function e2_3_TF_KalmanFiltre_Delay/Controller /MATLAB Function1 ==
function [theta,phi] = fcn(eax,eay)
g=9.8;

theta =-eax/g;% vx
phi =eay/g;% vy

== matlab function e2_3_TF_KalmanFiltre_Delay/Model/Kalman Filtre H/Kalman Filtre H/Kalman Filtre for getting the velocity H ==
function [Covariance_matrice,X_Kalmanfiltred] = fcn(Mesurement_Velocity)

% Persistent process for saving the last state and initilizing the variable
persistent P0_static;
if isempty(P0_static)
    P0_static=[0.1,0 0;0,0.1,0;0 0 0.1]; % the initilized matrice of estimated error
end

persistent Xkf_static;
if isempty(Xkf_static)
    Xkf_static=[0;0;0]; % the initilized state from Kalman Estimaton
end

% Determine the constants

% Simple time
Ts =0.01;

% Process Noise
p_var =0.05; % sigma
Q = eye(3)*p_var^2; % the covariance matrice of process noise
W=Q*randn(3,1);  % process noise

% Mesurement Noise
m_var = 0.01; % sigma
R = [m_var^2 ];  % the covariance matrice of mesurement noise
V=R*randn; % mesurement noise

% Observation matrice
H=[1 0 0];

% The indentity matrice
I=eye(3); 

% State Transition Martrix
A=[1 Ts 0.5*(Ts^2);0 1 Ts;0 0 1];

% Steady-State equation

% persistent X_real_static;
% if isempty(X_real_static)
%     X_real_static=[0;0]; % the initilized state from Kalman Estimaton
% end
% X_real_forward=X_real_static;
% X_real=A*X_real_forward+W;
% Mesurement_Velocity=H*(X_real)+V;
% X_real_static=X_real;    

%   Kalman Update process
    X_pre=A*Xkf_static; % State estimation
    P_pre=A*P0_static*A'+Q; % Covariance matrice estimation

    Kg=P_pre*H'*inv(H*P_pre*H'+R); % Kalman Gain calculation

    X_Kalmanfiltred=X_pre+Kg*(Mesurement_Velocity-H*X_pre); % State estimation update
    Covariance_matrice=(I-Kg*H)*P_pre; % Covariance matrice estimation update

% update the value of the persistent variable for iterating the Kalman process
P0_static=Covariance_matrice;
Xkf_static=X_Kalmanfiltred;

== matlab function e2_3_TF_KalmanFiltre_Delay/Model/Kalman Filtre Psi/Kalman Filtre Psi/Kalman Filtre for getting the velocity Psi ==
function [Covariance_matrice,X_Kalmanfiltred] = fcn(Mesurement_Velocity)

% Persistent process for saving the last state and initilizing the variable
persistent P0_static;
if isempty(P0_static)
    P0_static=[0.1,0 0;0,0.1,0;0 0 0.1]; % the initilized matrice of estimated error
end

persistent Xkf_static;
if isempty(Xkf_static)
    Xkf_static=[0;0;0]; % the initilized state from Kalman Estimaton
end

% Determine the constants

% Simple time
Ts =0.01;

% Process Noise
p_var =0.01; % sigma
Q = eye(3)*p_var^2; % the covariance matrice of process noise
W=Q*randn(3,1);  % process noise

% Mesurement Noise
m_var = 0.05; % sigma
R = [m_var^2 ];  % the covariance matrice of mesurement noise
V=R*randn; % mesurement noise

% Observation matrice
H=[1 0 0];

% The indentity matrice
I=eye(3); 

% State Transition Martrix
A=[1 Ts 0.5*(Ts^2);0 1 Ts;0 0 1];


% Steady-State equation

% persistent X_real_static;
% if isempty(X_real_static)
%     X_real_static=[0;0]; % the initilized state from Kalman Estimaton
% end
% X_real_forward=X_real_static;
% X_real=A*X_real_forward+W;
% Mesurement_Velocity=H*(X_real)+V;
% X_real_static=X_real;    

%   Kalman Update process
    X_pre=A*Xkf_static; % State estimation
    P_pre=A*P0_static*A'+Q; % Covariance matrice estimation

    Kg=P_pre*H'*inv(H*P_pre*H'+R); % Kalman Gain calculation

    X_Kalmanfiltred=X_pre+Kg*(Mesurement_Velocity-H*X_pre); % State estimation update
    Covariance_matrice=(I-Kg*H)*P_pre; % Covariance matrice estimation update

% update the value of the persistent variable for iterating the Kalman process
P0_static=Covariance_matrice;
Xkf_static=X_Kalmanfiltred;

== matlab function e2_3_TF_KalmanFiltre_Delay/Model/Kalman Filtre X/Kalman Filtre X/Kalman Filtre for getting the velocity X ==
function [Covariance_matrice,X_Kalmanfiltred] = fcn(Mesurement_Velocity)

% Persistent process for saving the last state and initilizing the variable
persistent P0_static;
if isempty(P0_static)
    P0_static=[0.1,0 0;0,0.1,0;0 0 0.1]; % the initilized matrice of estimated error
end

persistent Xkf_static;
if isempty(Xkf_static)
    Xkf_static=[0;0;0]; % the initilized state from Kalman Estimaton
end

% Determine the constants

% Simple time
Ts =0.01;

% Process Noise
p_var =0.05; % sigma
Q = eye(3)*p_var^2; % the covariance matrice of process noise
W=Q*randn(3,1);  % process noise

% Mesurement Noise
m_var = 0.01; % sigma
R = [m_var^2 ];  % the covariance matrice of mesurement noise
V=R*randn; % mesurement noise

% Observation matrice
H=[1 0 0];

% The indentity matrice
I=eye(3); 

% State Transition Martrix
A=[1 Ts 0.5*(Ts^2);0 1 Ts;0 0 1];

% Steady-State equation

% persistent X_real_static;
% if isempty(X_real_static)
%     X_real_static=[0;0]; % the initilized state from Kalman Estimaton
% end
% X_real_forward=X_real_static;
% X_real=A*X_real_forward+W;
% Mesurement_Velocity=H*(X_real)+V;
% X_real_static=X_real;    

%   Kalman Update process
    X_pre=A*Xkf_static; % State estimation
    P_pre=A*P0_static*A'+Q; % Covariance matrice estimation

    Kg=P_pre*H'*inv(H*P_pre*H'+R); % Kalman Gain calculation

    X_Kalmanfiltred=X_pre+Kg*(Mesurement_Velocity-H*X_pre); % State estimation update
    Covariance_matrice=(I-Kg*H)*P_pre; % Covariance matrice estimation update

% update the value of the persistent variable for iterating the Kalman process
P0_static=Covariance_matrice;
Xkf_static=X_Kalmanfiltred;

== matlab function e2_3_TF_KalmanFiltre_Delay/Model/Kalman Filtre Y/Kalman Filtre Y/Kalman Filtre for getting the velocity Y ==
function [Covariance_matrice,X_Kalmanfiltred] = fcn(Mesurement_Velocity)

% Persistent process for saving the last state and initilizing the variable
persistent P0_static;
if isempty(P0_static)
    P0_static=[0.1,0 0;0,0.1,0;0 0 0.1]; % the initilized matrice of estimated error
end

persistent Xkf_static;
if isempty(Xkf_static)
    Xkf_static=[0;0;0]; % the initilized state from Kalman Estimaton
end

% Determine the constants

% Simple time
Ts =0.01;

% Process Noise
p_var =0.05; % sigma
Q = eye(3)*p_var^2; % the covariance matrice of process noise
W=Q*randn(3,1);  % process noise

% Mesurement Noise
m_var =0.01; % sigma
R = [m_var^2 ];  % the covariance matrice of mesurement noise
V=R*randn; % mesurement noise

% Observation matrice
H=[1 0 0];

% The indentity matrice
I=eye(3); 

% State Transition Martrix
A=[1 Ts 0.5*(Ts^2);0 1 Ts;0 0 1];

% Steady-State equation

% persistent X_real_static;
% if isempty(X_real_static)
%     X_real_static=[0;0]; % the initilized state from Kalman Estimaton
% end
% X_real_forward=X_real_static;
% X_real=A*X_real_forward+W;
% Mesurement_Velocity=H*(X_real)+V;
% X_real_static=X_real;    

%   Kalman Update process
    X_pre=A*Xkf_static; % State estimation
    P_pre=A*P0_static*A'+Q; % Covariance matrice estimation

    Kg=P_pre*H'*inv(H*P_pre*H'+R); % Kalman Gain calculation

    X_Kalmanfiltred=X_pre+Kg*(Mesurement_Velocity-H*X_pre); % State estimation update
    Covariance_matrice=(I-Kg*H)*P_pre; % Covariance matrice estimation update

% update the value of the persistent variable for iterating the Kalman process
P0_static=Covariance_matrice;
Xkf_static=X_Kalmanfiltred;
